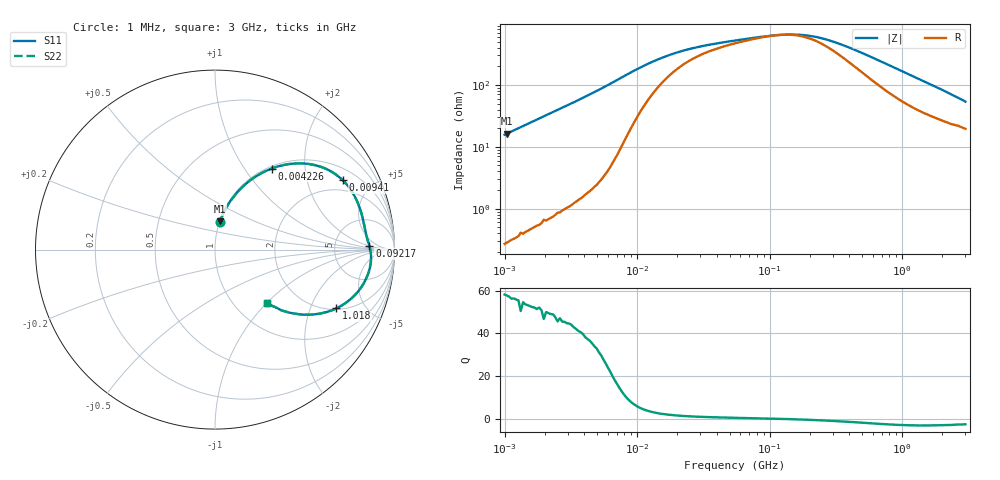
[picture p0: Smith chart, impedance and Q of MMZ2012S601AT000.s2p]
! S-parameter Generated by TDK Corporation
! Copyright(C) 2016 TDK Corporation.
! All Rights Reserved.
! TDK P/N: MMZ2012S601AT000 (Chip Beads)
! Property: |Z|=600¶ at 100MHz
! Size(LxWxT): 2x1.25x0.85mm, 0.079x0.049x0.033inches
! Model Type: s2p (Touchstone File Format Version 1.0)
! Frequency: DC=Yes Start=1MHz Stop=3000MHz 202points Log-sweep
! Note: This model was converted from impedance.
! Model Generated on May. 16, 2016
! Hash(MD5):
! Port Assignments:
!  1 ---@@@--- 2
! Applicable Conditions:
!  Temperature = 25 degC
!  DC Bias Current = 0 A
!  Small Signal Operation
! Terms and conditions regarding TDK Simulation Models
! (1)This simulation model is being provided solely for informational purposes. Please refer to the specifications of the products in terms of detailed characteristics of such products.
! (2)In no event shall TDK Corporation of any of its subsidiaries be liable for any loss or damage arising, directly or indirectly,
!  From any information contained in this simulation model, including, but not limited to loss or damages arising from any inaccuracies, omissions or errors in connection with such information.
! (3)Any and all copyrights on this simulation model are owned by TDK Corporation.
!  Duplication or redistribution of this simulation model without prior written permission from TDK Corporation is prohibited.
! (4)This simulation model is subject to any modification or change without any prior notice.
! (5)Neither TDK Corporation nor any of its subsidiaries shall make any warranty, express or implied,
!  Including but not limited to the correctness, implied warranties of merchantability and fitness for a particular purpose with respect to this simulation models.
! (6)The use of this simulation model shall be deemed to have consented to the terms and conditions hereof.
# MHz S MA R 50
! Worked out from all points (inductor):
!   201 points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, 1 MHz to 3 GHz, reference 50 ohm
!   read as one part in series: L = 2.49 uH near 1.041 MHz
!   highest Q = 57.7 at 1.041 MHz (marker M1), where L = 2.5 uH
!   self-resonance near 119.8 MHz
!   S11 on the Smith chart (normalised r, x): 1 MHz: 1.01, +0.31; 4.226 MHz: 1.04, +1.35; 9.41 MHz: 1.48, +3.33; 92.17 MHz: 13, +2; 1.018 GHz: 2.06, -3.09; 3 GHz: 1.39, -1.00
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1  0.1546 80.1  0.9853 -8.9  0.9853 -8.9  0.1546 80.1
1.040844  0.1607 79.8  0.9842 -9.2  0.9842 -9.2  0.1607 79.8
1.553251  0.2353 75.3  0.9675 -13.6  0.9675 -13.6  0.2353 75.3
2.226959  0.3272 69.7  0.9383 -19.1  0.9383 -19.1  0.3272 69.7
3.067588  0.4306 63.2  0.8929 -25.5  0.8929 -25.5  0.4306 63.2
3.900413  0.52 57.2  0.8412 -31.3  0.8412 -31.3  0.52 57.2
4.225536  0.5514 55.0  0.8196 -33.5  0.8196 -33.5  0.5514 55.0
6.305767  0.7077 42.4  0.6747 -45.0  0.6747 -45.0  0.7077 42.4
7.703107  0.7704 35.3  0.5795 -50.2  0.5795 -50.2  0.7704 35.3
9.410094  0.81 28.5  0.4821 -53.3  0.4821 -53.3  0.81 28.5
14.61624  0.838 17.3  0.3198 -51.3  0.3198 -51.3  0.838 17.3
25.59965  0.8424 9.4  0.218 -39.2  0.218 -39.2  0.8424 9.4
54.77226  0.8503 4.1  0.1633 -21.7  0.1633 -21.7  0.8503 4.1
92.16659  0.8603 1.4  0.1416 -8.6  0.1416 -8.6  0.8603 1.4
143.1579  0.868 -1.1  0.1331 7.0  0.1331 7.0  0.868 -1.1
213.6344  0.8712 -3.9  0.1436 24.4  0.1436 24.4  0.8712 -3.9
294.2768  0.8688 -6.7  0.171 36.6  0.171 36.6  0.8688 -6.7
439.1493  0.8559 -11.3  0.2326 46.3  0.2326 46.3  0.8559 -11.3
800.5644  0.796 -21.1  0.3847 48.0  0.3847 48.0  0.796 -21.1
1017.911  0.7512 -25.8  0.4604 45.3  0.4604 45.3  0.7512 -25.8
1712.864  0.6089 -36.5  0.6259 35.3  0.6259 35.3  0.6089 -36.5
3000  0.4142 -45.9  0.7716 22.7  0.7716 22.7  0.4142 -45.9
